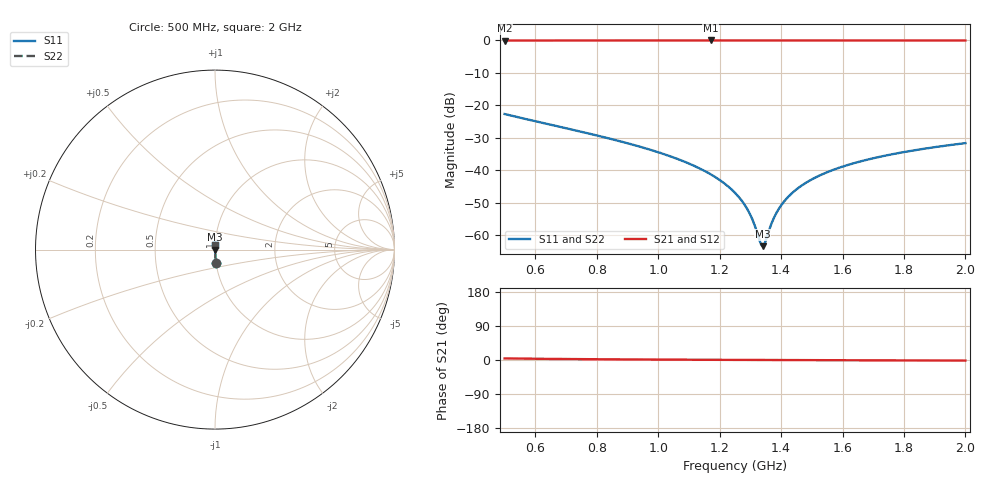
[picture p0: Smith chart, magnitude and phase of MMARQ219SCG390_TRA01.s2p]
! MMARQ219SCG390_TRA01  S-PARAMETER MODEL  ( General Type )
! Model Generated by TAIYO YUDEN Corporation (http://www.ty-top.com)
! Version 1.0
! TAIYO YUDEN Control No. 150609
! Copyright(c) 2015 TAIYO YUDEN CO.,LTD. All Rights Reserved.
! Product Description (link to TY-COMPAS)
! https://ds.yuden.co.jp/TYCOMPAS/or/detail?pn=MMARQ219SCG390JTRA01&u=M
! Products Name : Multilayer Ceramic Capacitors
! Characteristics :
!  Capacitance : 39 pF , Rated Voltage : 250V , TCC : CG / C0G
!  Case Size : 2.0 x 1.25 / 0.079 x 0.049 [mm/inch] , Thickness : 0.85 / 0.033 [mm/inch]
!  (Conditions: Temperature = 25 degC , DC Bias Current/Voltage = 0A / 0V)
! External Node Assignments :
!  1  o---| |---o  2
! GND o---------o GND
! Frequency Range : 500MHz  -  2GHz  [ 401 STEP ]
# MHz S RI R 50
! Freq[MHz].  S11 Real  S11 Imag  S21 Real  S21 Imag  S12 Real  S12 Imag  S22 Real  S22 Imag
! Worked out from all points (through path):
!   401 points, 500 MHz to 2 GHz, reference 50 ohm
!   highest |S21| = -0.01 dB at 1.171 GHz (marker M1); lowest = 0.0 dB at 500 MHz (marker M2)
!   lowest |S11| = -63.4 dB at 1.34 GHz (marker M3), VSWR 1.00, Z = 50.1 - j0.00105 ohm
!   |S11| at or under -10 dB: start of sweep to end of sweep
!   |S22| runs from -63.4 to -22.7 dB; largest |S21 - S12| = 0
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500  0.00573 -0.0733  0.9943 0.0733  0.9943 0.0733  0.00573 -0.0733
751.25  0.00193 -0.039  0.9981 0.039  0.9981 0.039  0.00193 -0.039
1002.5  0.000868 -0.0188  0.9991 0.0188  0.9991 0.0188  0.000868 -0.0188
1096.25  0.000724 -0.0129  0.9993 0.0129  0.9993 0.0129  0.000724 -0.0129
1171.25  0.000668 -0.00862  0.9993 0.00862  0.9993 0.00862  0.000668 -0.00862
1216.25  0.000653 -0.0062  0.9993 0.0062  0.9993 0.0062  0.000653 -0.0062
1250  0.000651 -0.00445  0.9993 0.00445  0.9993 0.00445  0.000651 -0.00445
1276.25  0.000654 -0.00312  0.9993 0.00312  0.9993 0.00312  0.000654 -0.00312
1295  0.000659 -0.00219  0.9993 0.00219  0.9993 0.00219  0.000659 -0.00219
1310  0.000664 -0.00145  0.9993 0.00145  0.9993 0.00145  0.000664 -0.00145
1332.5  0.000674 -0.000368  0.9993 0.000368  0.9993 0.000368  0.000674 -0.000368
1340  0.000677 -1.05e-05  0.9993 1.05e-05  0.9993 1.05e-05  0.000677 -1.05e-05
1347.5  0.000681 0.000345  0.9993 -0.000345  0.9993 -0.000345  0.000681 0.000345
1366.25  0.000692 0.00123  0.9993 -0.00123  0.9993 -0.00123  0.000692 0.00123
1377.5  0.0007 0.00175  0.9993 -0.00175  0.9993 -0.00175  0.0007 0.00175
1403.75  0.00072 0.00295  0.9993 -0.00295  0.9993 -0.00295  0.00072 0.00295
1445  0.000756 0.0048  0.9992 -0.0048  0.9992 -0.0048  0.000756 0.0048
1501.25  0.000817 0.00724  0.9992 -0.00724  0.9992 -0.00724  0.000817 0.00724
1550  0.000878 0.00929  0.9991 -0.00929  0.9991 -0.00929  0.000878 0.00929
1606.25  0.000959 0.0116  0.999 -0.0116  0.999 -0.0116  0.000959 0.0116
1752.5  0.00121 0.0173  0.9988 -0.0173  0.9988 -0.0173  0.00121 0.0173
2000  0.00176 0.0261  0.9982 -0.0261  0.9982 -0.0261  0.00176 0.0261
